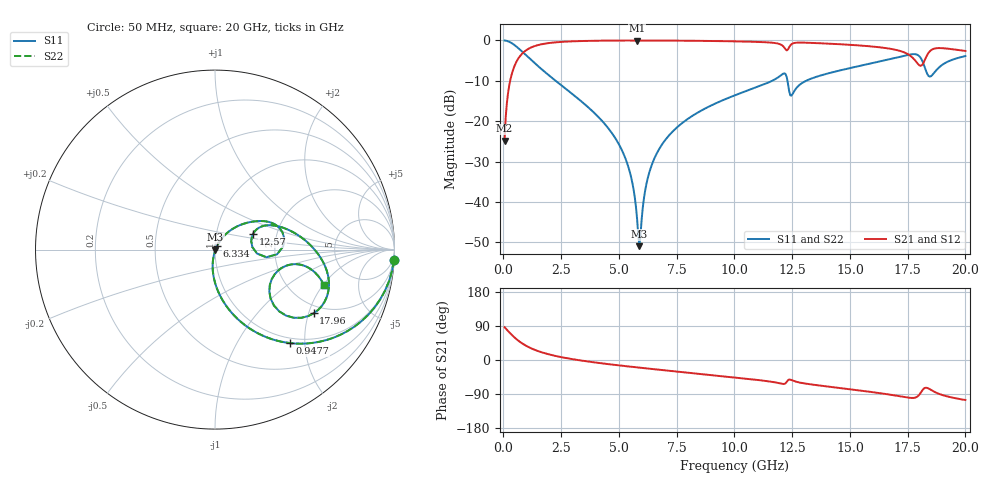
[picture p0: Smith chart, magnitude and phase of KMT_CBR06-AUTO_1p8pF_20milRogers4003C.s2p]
! Data measured by Modelithics Inc. support@modelithics.com 813-866-6335
! KEMET CBR06-AUTO 1.8pF, Pad Width= 0.851mm, Pad Length= 0.64mm, Pad Gap= 0.62mm, 20mil Rogers 4003C substrate Data, January 2022
# hz S ma R 50
! 2 Port Network Data from SP1.SP block
! freq  magS11  angS11  magS21  angS21  magS12  angS12  magS22  angS22
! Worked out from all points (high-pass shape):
!   401 points, 50 MHz to 20 GHz, reference 50 ohm
!   highest |S21| = -0.03 dB at 5.786 GHz (marker M1); lowest = -24.9 dB at 50 MHz (marker M2)
!   |S21| within 3 dB of the highest: 855.7 MHz to 17.37 GHz (16.52 GHz wide, 181 % of centre); 18.41 GHz to end of sweep
!   lowest |S11| = -51.0 dB at 5.885 GHz (marker M3), VSWR 1.01, Z = 50.3 - j0.098 ohm
!   |S11| at or under -10 dB: 2.259 GHz to 11.63 GHz (9.376 GHz wide, 135 % of centre); 12.29 GHz to 13.11 GHz (810.5 MHz wide, 6.38 % of centre)
!   |S22| runs from -51.0 to 0.0 dB; largest |S21 - S12| = 0
!   S11 on the Smith chart (normalised r, x): 50 MHz: 1, -33; 947.8 MHz: 0.91, -1.71; 6.334 GHz: 1.02, +0.04; 12.57 GHz: 1.51, +0.28; 17.96 GHz: 1.74, -2.16; 20 GHz: 3.05, -2.06
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5e7  0.9984 -3.4  0.05714 86.5  0.05714 86.5  0.9984 -3.4
3.4925e8  0.9279 -23.0  0.3721 66.9  0.3721 66.9  0.9279 -23.0
9.4775e8  0.6683 -51.2  0.7425 38.7  0.7425 38.7  0.6683 -51.2
1.8455e9  0.3947 -72.8  0.9169 16.9  0.9169 16.9  0.3947 -72.8
3.391625e9  0.1739 -90.9  0.9823 -1.7  0.9823 -1.7  0.1739 -90.9
5.13725e9  0.04314 -101.6  0.9962 -15.2  0.9962 -15.2  0.04314 -101.6
5.53625e9  0.01973 -99.8  0.9969 -17.9  0.9969 -17.9  0.01973 -99.8
5.785625e9  0.006171 -82.4  0.997 -19.5  0.997 -19.5  0.006171 -82.4
5.885375e9  0.00283 -20.1  0.997 -20.2  0.997 -20.2  0.00283 -20.1
6.33425e9  0.02421 60.0  0.9966 -23.1  0.9966 -23.1  0.02421 60.0
6.73325e9  0.04473 60.5  0.9958 -25.6  0.9958 -25.6  0.04473 60.5
7.93025e9  0.1041 55.1  0.991 -33.0  0.991 -33.0  0.1041 55.1
1.0025e10  0.2092 42.7  0.9733 -46.1  0.9733 -46.1  0.2092 42.7
1.211975e10  0.388 14.4  0.8412 -63.2  0.8412 -63.2  0.388 14.4
1.231925e10  0.2896 -8.5  0.7732 -53.3  0.7732 -53.3  0.2896 -8.5
1.256862e10  0.2298 22.5  0.9258 -55.3  0.9258 -55.3  0.2298 22.5
1.336662e10  0.3398 23.6  0.9304 -64.8  0.9304 -64.8  0.3398 23.6
1.670825e10  0.5817 -3.3  0.791 -91.2  0.791 -91.2  0.5817 -3.3
1.795512e10  0.6544 -32.9  0.5077 -94.8  0.5077 -94.8  0.6544 -32.9
1.845388e10  0.3565 -27.4  0.7299 -76.8  0.7299 -76.8  0.3565 -27.4
1.885288e10  0.4611 -10.1  0.8038 -89.3  0.8038 -89.3  0.4611 -10.1
2e10  0.6395 -18.1  0.7401 -105.6  0.7401 -105.6  0.6395 -18.1
